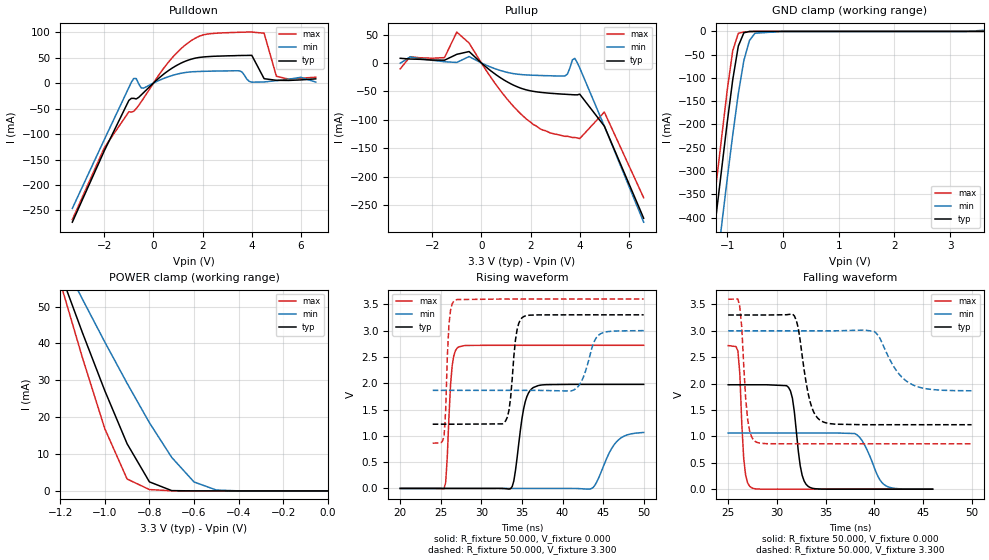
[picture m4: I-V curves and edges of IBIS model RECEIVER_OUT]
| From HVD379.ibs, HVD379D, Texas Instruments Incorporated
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[Model]   RECEIVER_OUT
Model_type   Output
| Signals   R
Vmeas = 1.3V   |Reference voltage for timing measurements
Cref = 15pF   |Timing specification test load capacitance value
| variable   typ   min   max
C_comp   25pF   20pF   30pF
|   typ   min   max
[Temperature Range]   25.0   -40   85
[Voltage range]   3.3V   3.0V   3.6V
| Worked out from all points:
|   slope of the pulldown table from 0 to 0.495 V, typ, clamps not added: 24.2 ohm
|   slope of the pullup table from 0 to 0.495 V, typ, clamps not added: 28.4 ohm
|   GND clamp passes 1 mA (typ) near -0.63 V on its own axis
|   POWER clamp passes 1 mA (typ) near -0.74 V on its own axis
|   rising waveform, R_fixture 50.000, V_fixture 0.000: 20-80 % time 1.06ns typ, 1.98ns min, 539ps max; typ from 0 V to 1.98 V
|   falling waveform, R_fixture 50.000, V_fixture 0.000: 20-80 % time 745ps typ, 1.5ns min, 417ps max; typ from 1.98 V to 0 V
|   rising waveform, R_fixture 50.000, V_fixture 3.300: 20-80 % time 735ps typ, 1.35ns min, 416ps max; typ from 1.22 V to 3.3 V
|   falling waveform, R_fixture 50.000, V_fixture 3.300: 20-80 % time 1.11ns typ, 2.21ns min, 556ps max; typ from 3.3 V to 1.22 V
[Pulldown]
|   Voltage   I(typ)   I(min)   I(max)
-3.3V     -273mA     -246mA     -268mA
-2V       -133mA     -111mA     -127mA
-1V       -34mA      -8.7mA     -56.3mA
-800mV    -30mA      9.09mA     -55.4mA
-400mV    -18.7mA    -9.91mA    -29.7mA
700mV     27.4mA     13.9mA     46.2mA
1.6V      47.7mA     22.2mA     85.2mA
3.5V      54mA       24mA       99.6mA
4V        54.3mA     1.69mA     100mA
4.5V      8.57mA     2.13mA     97.8mA
5V        5.36mA     4.73mA     13.3mA
6.6V      8.22mA     1.9mA      11.4mA
[Pullup]
|   Voltage   I(typ)   I(min)   I(max)
| Note that the[Pullup]voltage table is referenced to Vcc
| and is calculated using Vtable=Vcc - Vmeasured.
-3.3V     8.22mA     -444uA     -10.4mA
-2.9V     6.92mA     10.7mA     11mA
-1.5V     4.87mA     2.13mA     9.41mA
-1V       15.2mA     886uA      54.3mA
-500mV    20.1mA     11.3mA     35mA
700mV     -23.8mA    -12.2mA    -44.3mA
1.8V      -47mA      -20.9mA    -97.4mA
3.4V      -55mA      -22.7mA    -129mA
3.8V      -56mA      8.09mA     -131mA
4V        -54.9mA    -8.7mA     -133mA
5V        -111mA     -111mA     -86.3mA
6.6V      -273mA     -280mA     -237mA
[GND_clamp]
|   Voltage   I(typ)   I(min)   I(max)
-3.6V     -2.758A    -2.85A     -2.739A
-1.5V     -698.7mA   -815.7mA   -635.9mA
-1V       -197mA     -318.3mA   -127.7mA
-900mV    -104mA     -222.6mA   -41.44mA
-800mV    -31.56mA   -134.1mA   -4.066mA
-700mV    -2.903mA   -62.37mA   -1.291mA
-600mV    -136.4uA   -19.38mA   -399.1uA
-500mV    -7.538uA   -3.856mA   -41.25uA
0V        -39.6pA    -277.7pA   -43.2pA
3.3V      43.52pA    1.004uA    41.74pA
3.6V      70.17pA    2.426mA    48.41pA
[POWER_clamp]
|   Voltage  I(typ)   I(min)   I(max)
| Note that the [POWER_clamp] voltage table is referenced to Vcc
| and is calculated using Vtable = Vcc - Vmeasured.
| Outputs in Tri-state.
-3.3V     426mA      323mA      525mA
-1.2V     59.3mA     63.8mA     56.7mA
-1.1V     42.9mA     52mA       36.1mA
-1V       27.2mA     40.4mA     16.9mA
-900mV    12.8mA     29.2mA     3.23mA
-800mV    2.46mA     18.5mA     371uA
-700mV    85.9uA     9.09mA     34.2uA
-600mV    1.86uA     2.43mA     1.25uA
-500mV    40.3nA     243uA      23.5nA
-400mV    931pA      16uA       387pA
0V        43.5pA     6.39nA     48.4pA
[Ramp]
|   typ   min   max
dV/dt_r   1.25V/865ps   0.665V/1997ps   1.64V/384ps
dV/dt_f   1.25V/1107ps   0.753V/2223ps   1.63V/417ps
R_load = 50
[Rising Waveform]
R_fixture = 50.000
V_fixture = 0.000
C_fixture = 0.000
L_fixture = 0.000
|  time   V(typ)   V(min)   V(max)
20ns      50.21nV    1.391nV    38.12nV
25.4ns    50.26nV    1.391nV    -6.057mV
26.4ns    50.22nV    1.391nV    2.331V
27.2ns    50.71nV    1.343nV    2.691V
33.8ns    36.42mV    8.888nV    2.721V
35.2ns    1.508V     38.74nV    2.721V
36.4ns    1.918V     31.91nV    2.721V
43.6ns    1.978V     -647uV     2.721V
46.6ns    1.978V     876.3mV    2.721V
50ns      1.978V     1.064V     2.721V
[Falling Waveform]
R_fixture = 50.000
V_fixture = 0.000
C_fixture = 0.000
L_fixture = 0.000
|  time   V(typ)   V(min)   V(max)
25ns      1.978V     1.064V     2.721V
26ns      1.978V     1.064V     2.621V
26.6ns    1.978V     1.064V     572.7mV
27.4ns    1.978V     1.064V     26.46mV
31.2ns    1.928V     1.064V     717nV
32.6ns    262.9mV    1.064V     141nV
33.4ns    33.05mV    1.064V     101.6nV
38ns      11.46uV    1.054V     54.89nV
41ns      371.3nV    89.2mV     47.77nV
46ns      90.22nV    1.391nV    42.97nV
[Rising Waveform]
R_fixture = 50.000
V_fixture = 3.300
V_fixture_min = 3.000
V_fixture_max = 3.600
C_fixture = 0.000
L_fixture = 0.000
|  time   V(typ)   V(min)   V(max)
24ns      1.221V     1.864V     859.6mV
25.4ns    1.221V     1.864V     987.4mV
26ns      1.221V     1.864V     3.106V
26.8ns    1.221V     1.864V     3.582V
33ns      1.287V     1.864V     3.6V
34.4ns    3.018V     1.864V     3.6V
35.2ns    3.266V     1.864V     3.6V
41.4ns    3.3V       1.873V     3.6V
44.4ns    3.3V       2.907V     3.6V
50ns      3.3V       3V         3.6V
[Falling Waveform]
R_fixture = 50.000
V_fixture = 3.300
V_fixture_min = 3.000
V_fixture_max = 3.600
C_fixture = 0.000
L_fixture = 0.000
|  time   V(typ)   V(min)   V(max)
25ns      3.3V       3V         3.6V
26.2ns    3.3V       3V         3.45V
27ns      3.3V       3V         1.325V
27.8ns    3.3V       3V         901.2mV
31.8ns    3.283V     3V         859.6mV
33.4ns    1.666V     3V         859.6mV
34.6ns    1.288V     3V         859.6mV
40ns      1.221V     2.989V     859.6mV
43.6ns    1.221V     2.012V     859.6mV
50ns      1.221V     1.864V     859.6mV
